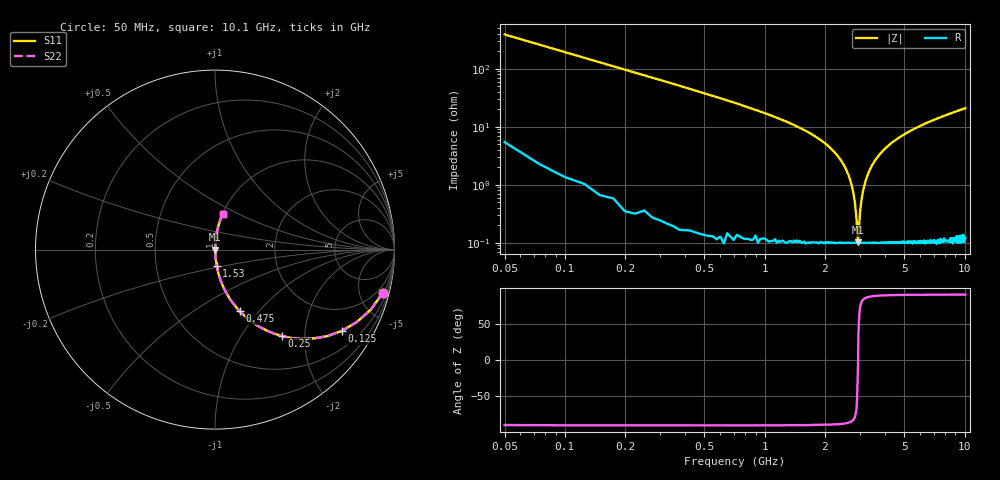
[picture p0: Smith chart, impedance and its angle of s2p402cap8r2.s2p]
! AVX Thin Film Operation		Date: April 2003
! Description: Accu-P® Series, Thin Film, SMD, RF Capacitor
! Part Number: 0402ZK8R2BBW
! 50 MHz  -  10.05 GHz
! Serial Measurements
# hz S db R 50
!	S11		S21		S12		S22
!	dB	Phase	dB	Phase	dB	Phase	dB	Phase
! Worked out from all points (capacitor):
!   400 points, 50 MHz to 10.1 GHz, reference 50 ohm
!   read as one part in series: C = 8.2 pF near 100 MHz
!   lowest |Z| = 102 mohm at 2.93 GHz (marker M1)
!   series resonance near 2.933 GHz, so ESL is about 360 pH
!   S11 on the Smith chart (normalised r, x): 50 MHz: 1.10, -7.76; 125 MHz: 1.02, -3.10; 250 MHz: 1.01, -1.54; 475 MHz: 1.00, -0.80; 1.53 GHz: 1.00, -0.19; 10.1 GHz: 1.00, +0.42
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5e7  -0.31 -14.4  -12.10 74.8  -12.10 74.8  -0.31 -14.4
1.25e8  -1.53 -32.7  -5.34 56.9  -5.34 56.9  -1.53 -32.7
2.5e8  -4.30 -52.2  -2.04 37.5  -2.04 37.5  -4.30 -52.2
4.75e8  -8.65 -68.1  -0.65 21.7  -0.65 21.7  -8.65 -68.1
9e8  -14.40 -78.6  -0.17 11.0  -0.17 11.0  -14.40 -78.6
1.53e9  -20.70 -84.1  -0.05 5.3  -0.05 5.3  -20.70 -84.1
1.73e9  -22.70 -85.0  -0.03 4.2  -0.03 4.2  -22.70 -85.0
2.28e9  -29.40 -86.4  -0.01 1.9  -0.01 1.9  -29.40 -86.4
2.63e9  -36.70 -85.2  -0.01 0.8  -0.01 0.8  -36.70 -85.2
2.73e9  -40.30 -83.5  -0.01 0.5  -0.01 0.5  -40.30 -83.5
2.83e9  -46.20 -78.0  -0.01 0.3  -0.01 0.3  -46.20 -78.0
2.88e9  -51.50 -67.9  -0.01 0.1  -0.01 0.1  -51.50 -67.9
2.93e9  -59.80 -11.0  -0.01 0.0  -0.01 0.0  -59.80 -11.0
3e9  -49.60 72.3  -0.01 -0.2  -0.01 -0.2  -49.60 72.3
3.1e9  -42.40 82.0  -0.01 -0.4  -0.01 -0.4  -42.40 82.0
3.25e9  -37.20 85.1  -0.01 -0.8  -0.01 -0.8  -37.20 85.1
3.4e9  -34.10 86.0  -0.01 -1.1  -0.01 -1.1  -34.10 86.0
4.05e9  -27.20 86.2  -0.02 -2.5  -0.02 -2.5  -27.20 86.2
5.08e9  -22.40 84.9  -0.03 -4.4  -0.03 -4.4  -22.40 84.9
6.75e9  -18.20 82.5  -0.08 -7.1  -0.08 -7.1  -18.20 82.5
8.43e9  -15.60 80.1  -0.13 -9.5  -0.13 -9.5  -15.60 80.1
1.01e10  -13.80 77.9  -0.19 -11.7  -0.19 -11.7  -13.80 77.9
